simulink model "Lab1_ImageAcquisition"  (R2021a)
settings: Solver=ode4  StartTime=0.0  StopTime=inf  FixedStep=1/30  RelTol=1e-3  EnableMultiTasking=on
undefined symbols (not defined in the file): HxWx3, imread, MATLAB, RGB, Video3D, x
libraries: quarc_library x17

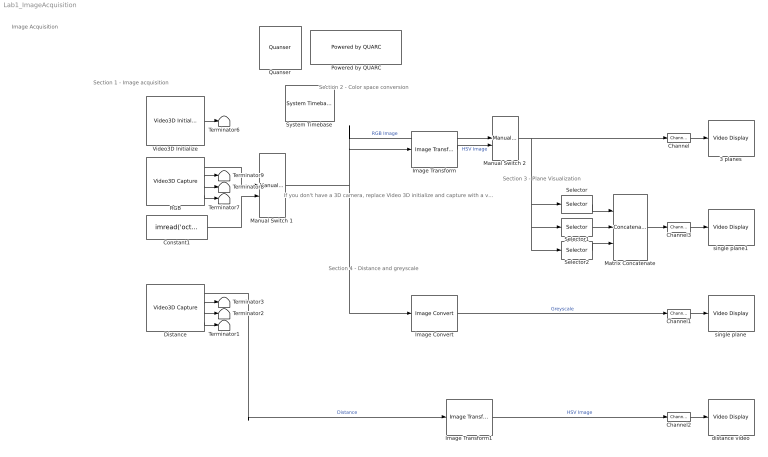
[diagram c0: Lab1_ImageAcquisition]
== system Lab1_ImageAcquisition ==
  note: If you don't have a 3D camera, replace Video 3D initialize and capture with a video capture block. (Delete bottom part ofsection 4 which shows distance image and it is not available) Manual switches will allow you to visualize the image in RGB/HSV and its three corresponding planes. The signel plane display in section 4 shows the greyscale image of the camera.
  note: Section 4 - Distance and greyscale
  note: Section 3 - Plane Visualization
  note: Section 2 - Color space conversion
  note: Image Acquisition
  note: Section 1 - Image acquisition
  3 planes : quarc_library/Multimedia/Video Display  Tag=Lab1_ImageAcquisition/3 planes  sample_time=-1  use_hardware=on
  Channel : quarc_library/Signal Routing/Channel  channel=0  buffer_size=1
  Channel1 : quarc_library/Signal Routing/Channel  channel=1  buffer_size=1
  Channel2 : quarc_library/Signal Routing/Channel  channel=2  buffer_size=1
  Channel3 : quarc_library/Signal Routing/Channel  channel=3  buffer_size=1
  Constant1 : Constant  Value=imread('octopus.jpg');
  Distance : quarc_library/Multimedia/Video3D Capture  object_name=Video3D-1  stream_type=Depth  stream_index=0  resolution=640 x 480  width=640  height=480  output_format=Distance in meters (HxW)  data_type=single  sample_time=qc_get_step_size  camera_intrinsics=off  depth_scale=off  brightness_override=off  brightness=50.0  contrast_override=off  contrast=50.0  hue_override=off  hue=50.0  saturation_override=off  saturation=50.0  sharpness_override=off  sharpness=50.0  gamma_override=off  gamma=50.0  gain_override=off  gain=50.0  backlightcompensation_override=off  backlightcompensation=50.0  whitebalance_override=Automatic white balance  whitebalance=50.0  exposure_override=Automatic exposure  exposure=30.0  emitter=Enable laser emitter  preset=Do not set camera presets
  Image Convert : quarc_library/Image Processing/Generic/Image Convert  input_format=MATLAB RGB (HxWx3)  padding=0  output_format=MATLAB greyscale (HxW)  data_type=uint8
  Image Transform : quarc_library/Image Processing/Generic/Image Transform  algorithm=RGB to HSV  color_theme=KRYGCBMW  min_pixel=0  max_pixel=4000  focal_length=308  principal_point=[262 334]  radial_coeffs=[-0.3129 0.0907]  tangential_coeffs=[]  extrapolated_pixel=0  interpolation=nearest  row_coords=0  column_coords=0  output_height=480  output_width=640  angle=0  origin=[240 320]  output_origin=[240 320]  output_data_type=uint8
  Image Transform1 : quarc_library/Image Processing/Generic/Image Transform  algorithm=Colorize  color_theme=KRYGCBMW  min_pixel=.2  max_pixel=3  focal_length=308  principal_point=[262 334]  radial_coeffs=[-0.3129 0.0907]  tangential_coeffs=[]  extrapolated_pixel=0  interpolation=nearest  row_coords=0  column_coords=0  output_height=480  output_width=640  angle=0  origin=[240 320]  output_origin=[240 320]  output_data_type=uint8
  Manual Switch 1 : ManualSwitch
  Manual Switch 2 : ManualSwitch
  Matrix Concatenate : Concatenate  NumInputs=3  Mode=Multidimensional array  ConcatenateDimension=2
  Powered by QUARC : quarc_library/Logos/Powered by QUARC
  Quanser : quarc_library/Logos/Quanser
  RGB : quarc_library/Multimedia/Video3D Capture  object_name=Video3D-1  stream_type=RGB  stream_index=0  resolution=640 x 480  width=640  height=480  output_format=MATLAB RGB (HxWx3)  data_type=uint8  sample_time=qc_get_step_size  camera_intrinsics=off  depth_scale=off  brightness_override=off  brightness=50.0  contrast_override=off  contrast=50.0  hue_override=off  hue=50.0  saturation_override=off  saturation=50.0  sharpness_override=off  sharpness=50.0  gamma_override=off  gamma=50.0  gain_override=off  gain=50.0  backlightcompensation_override=off  backlightcompensation=50.0  whitebalance_override=Automatic white balance  whitebalance=50.0  exposure_override=Automatic exposure  exposure=30.0  emitter=Enable laser emitter  preset=Do not set camera presets
  Selector : Selector  NumberOfDimensions=3  InputPortWidth=3  IndexOptions=Select all,Select all,Index vector (dialog)  Indices=[1 3],1,1  OutputSizes=1,1,1
  Selector1 : Selector  NumberOfDimensions=3  InputPortWidth=3  IndexOptions=Select all,Select all,Index vector (dialog)  Indices=[1 3],1,2  OutputSizes=1,1,1
  Selector2 : Selector  NumberOfDimensions=3  InputPortWidth=3  IndexOptions=Select all,Select all,Index vector (dialog)  Indices=[1 3],1,3  OutputSizes=1,1,1
  System Timebase : quarc_library/Advanced/Timing/System Timebase  stop_on_overrun=off
  Terminator{1..3,6..9} (7 alike) : Terminator
  Video3D Initialize : quarc_library/Multimedia/Video3D Initialize  object_name=Video3D-1  source=Device  identifier=0  file=sample.bag  sample_time=qc_get_step_size  active=on
  distance video : quarc_library/Multimedia/Video Display  Tag=Lab1_ImageAcquisition/distance video  sample_time=-1  use_hardware=on
  single plane : quarc_library/Multimedia/Video Display  Tag=Lab1_ImageAcquisition/single plane  sample_time=-1  use_hardware=on
  single plane1 : quarc_library/Multimedia/Video Display  Tag=Lab1_ImageAcquisition/single plane1  sample_time=-1  use_hardware=on
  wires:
  RGB/3 -> Terminator8/1
  Video3D Initialize/1 -> Terminator6/1
  RGB/4 -> Terminator7/1
  RGB/2 -> Terminator9/1
  Channel/1 -> 3 planes/1
  Distance/2 -> Terminator3/1
  Distance/3 -> Terminator2/1
  Distance/4 -> Terminator1/1
  Distance/1 -> Image Transform1/1  "Distance"
  Channel1/1 -> single plane/1
  Channel2/1 -> distance video/1
  Image Transform/1 -> Manual Switch 2/2  "HSV Image"
  Image Transform1/1 -> Channel2/1  "HSV Image"
  Manual Switch 1/1 -> Manual Switch 2/1, Image Transform/1, Image Convert/1  "RGB Image"
  Image Convert/1 -> Channel1/1  "Greyscale"
  Manual Switch 2/1 -> Channel/1, Selector/1, Selector1/1, Selector2/1
  RGB/1 -> Manual Switch 1/1
  Channel3/1 -> single plane1/1
  Selector/1 -> Matrix Concatenate/1
  Selector1/1 -> Matrix Concatenate/2
  Selector2/1 -> Matrix Concatenate/3
  Matrix Concatenate/1 -> Channel3/1
  Constant1/1 -> Manual Switch 1/2
